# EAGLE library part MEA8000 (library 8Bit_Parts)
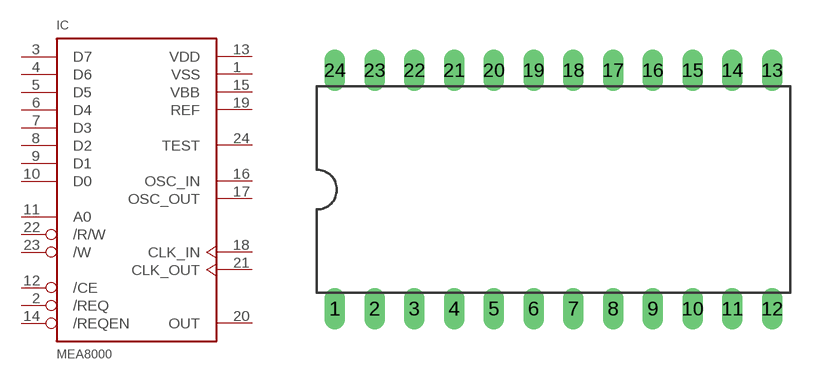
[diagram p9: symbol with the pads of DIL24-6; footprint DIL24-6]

Designator prefix IC

## MEA8000  [DIL24-6]
1  VSS  pwr
2  /REQ  in
3  D7  in
4  D6  in
5  D5  in
6  D4  in
7  D3  in
8  D2  in
9  D1  in
10  D0  in
11  A0  in
12  /CE  in
13  VDD  pwr
14  /REQEN  in
15  VBB  pwr
16  OSC_IN  in
17  OSC_OUT  out
18  CLK_IN  in
19  REF  in
20  OUT  out
21  CLK_OUT  out
22  /R/W  in
23  /W  in
24  TEST

## Footprint DIL24-6 (pad centres in mm)
Dual In Line Package 0.6 inch
drill 0.813 long: 1 -13.97,-7.62; 2 -11.43,-7.62; 3 -8.89,-7.62; 4 -6.35,-7.62; 5 -3.81,-7.62; 6 -1.27,-7.62; 7 1.27,-7.62; 8 3.81,-7.62; 9 6.35,-7.62; 10 8.89,-7.62; 11 11.43,-7.62; 12 13.97,-7.62; 13 13.97,7.62; 14 11.43,7.62; 15 8.89,7.62; 16 6.35,7.62; 17 3.81,7.62; 18 1.27,7.62; 19 -1.27,7.62; 20 -3.81,7.62; 21 -6.35,7.62; 22 -8.89,7.62; 23 -11.43,7.62; 24 -13.97,7.62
